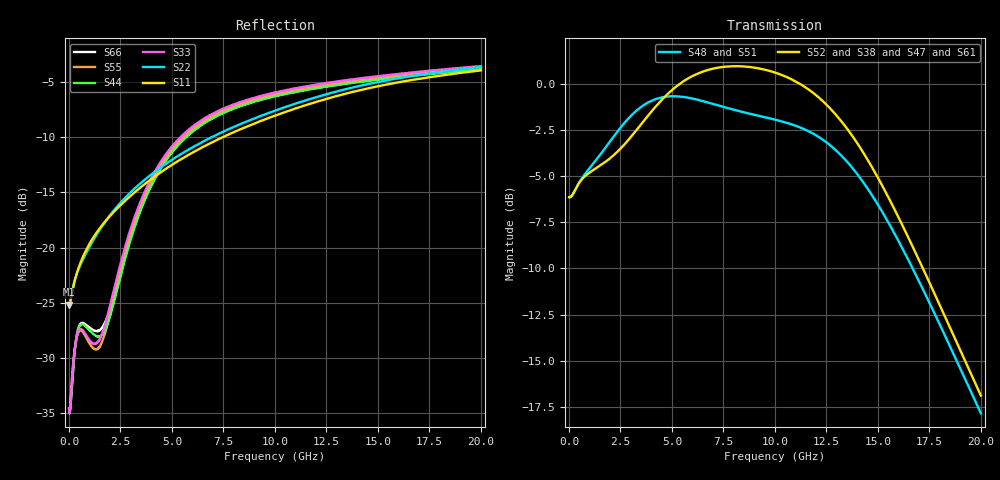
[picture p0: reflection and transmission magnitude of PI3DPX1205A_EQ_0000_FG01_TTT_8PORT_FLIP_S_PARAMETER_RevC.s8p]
! NPort=8 DATA=2000 NOISE=0 GROUPDELAY=0 COMPLEX_DATAFORMAT=POLAR
! NumOfBlock=1 NumOfParam=0
! .MODEL Smodel S TSTONEFILE=PI3DPX1205A_EQ_0000_FG01_TTT_8PORT_FLIP_S_PARAMETER_RevC.s8p TYPE=S
!  -- The above .MODEL line can be used for the S element in the netlist.
! The s parameter is extracted from the linear redriver, it is not bi-directional;
! only s(5,1)s(6,2)s(3,7)s(4,8) should be the insertion loss
!  Port definition:
!  Port1 = AIP
!  Port2 = AIN
!  Port3 = BOP
!  Port4 = BON
!  Port5 = AOP
!  Port6 = AON
!  Port7 = BIP
!  Port8 = BIN
# Hz S MA R  50
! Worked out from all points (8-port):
!   2000 points, 10 MHz to 20 GHz, reference 50 ohm
!   strongest paths, dB at 10 MHz, 5.01 GHz, 10.01 GHz, 15.01 GHz, 20 GHz:
!     S52: -6.1, -0.3, 0.6, -5.1, -16.9
!     S38: -6.1, -0.4, 0.6, -5.1, -16.9
!     S47: -6.1, -0.4, 0.6, -5.1, -16.8
!     S61: -6.1, -0.4, 0.6, -5.1, -16.8
!     S48: -6.1, -0.7, -2.0, -6.6, -17.8
!     S51: -6.1, -0.7, -2.0, -6.6, -17.8
!   lowest |S11| = -25.2 dB at 10 MHz (marker M1), VSWR 1.12, Z = 44.8 - j0.115 ohm
!   |S11| at or under -10 dB: start of sweep to 7.47 GHz
